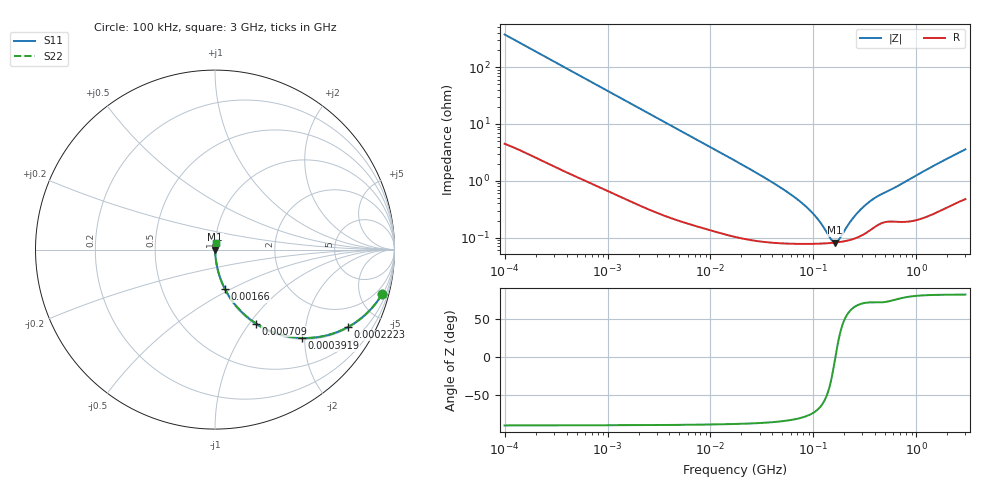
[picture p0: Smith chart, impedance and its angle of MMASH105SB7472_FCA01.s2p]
! MMASH105SB7472_FCA01  S-PARAMETER MODEL  ( Standard Model )
! Model Generated by TAIYO YUDEN Corporation (http://www.ty-top.com)
! Version 1.0
! TAIYO YUDEN Control No. 220601
! Copyright(c) 2019 TAIYO YUDEN CO.,LTD. All Rights Reserved.
! Product Description (link to TY-COMPAS)
! https://ds.yuden.co.jp/TYCOMPAS/or/detail?pn=MMASH105SB7472KFCA01&u=M
! Products Name : Multilayer Ceramic Capacitors
! Characteristics :
!  Capacitance : 4700 [pF] , Rated Voltage : 100 [V] , TCC : X7R
!  Case Size : 1.0 x 0.5 / 0.039 x 0.02 [mm/inch] , Thickness : 0.5 / 0.02 [mm/inch]
!  (Conditions: Temperature = 25 [degC] , DC Bias Voltage = 0 [V])
! External Node Assignments :
!  1  o---| |---o  2
! GND o---------o GND
! Frequency Range : 100kHz  -  3GHz  [ 401 STEP ]
# MHZ S RI R 50
! Freq[MHz].  S11 Real  S11 Imag  S21 Real  S21 Imag  S12 Real  S12 Imag  S22 Real  S22 Imag
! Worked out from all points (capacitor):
!   401 points, 100 kHz to 3 GHz, reference 50 ohm
!   read as one part in series: C = 4.23 nF near 105.3 kHz
!   lowest |Z| = 81.9 mohm at 163.1 MHz (marker M1)
!   series resonance near 163.6 MHz, so ESL is about 220 pH
!   S11 on the Smith chart (normalised r, x): 100 kHz: 1.09, -7.50; 222.3 kHz: 1.05, -3.40; 391.9 kHz: 1.03, -1.94; 709 kHz: 1.02, -1.08; 1.66 MHz: 1.01, -0.46; 3 GHz: 1.01, +0.07
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0.1  0.9311 -0.2474  0.0689 0.2474  0.0689 0.2474  0.9311 -0.2474
0.151038  0.8582 -0.3424  0.1418 0.3424  0.1418 0.3424  0.8582 -0.3424
0.222319  0.74 -0.4319  0.26 0.4319  0.26 0.4319  0.74 -0.4319
0.391939  0.4844 -0.4924  0.5156 0.4924  0.5156 0.4924  0.4844 -0.4924
0.562235  0.3173 -0.4577  0.6827 0.4577  0.6827 0.4577  0.3173 -0.4577
0.709011  0.2285 -0.4118  0.7715 0.4118  0.7715 0.4118  0.2285 -0.4118
1.043626  0.1232 -0.32  0.8768 0.32  0.8768 0.32  0.1232 -0.32
1.659646  0.0548 -0.2184  0.9452 0.2184  0.9452 0.2184  0.0548 -0.2184
3.161081  0.0173 -0.1202  0.9827 0.1202  0.9827 0.1202  0.0173 -0.1202
17.7727  0.0015 -0.0219  0.9985 0.0219  0.9985 0.0219  0.0015 -0.0219
53.83243  0.00083 -0.00658  0.9992 0.00658  0.9992 0.00658  0.00083 -0.00658
75.25761  0.000793 -0.00417  0.9992 0.00417  0.9992 0.00417  0.000793 -0.00417
97.38194  0.000784 -0.00264  0.9992 0.00264  0.9992 0.00264  0.000784 -0.00264
116.6348  0.000787 -0.00168  0.9992 0.00168  0.9992 0.00168  0.000787 -0.00168
147.0833  0.000804 -0.000521  0.9992 0.000521  0.9992 0.000521  0.000804 -0.000521
163.0551  0.000818 -1.6e-05  0.9992 1.6e-05  0.9992 1.6e-05  0.000818 -1.6e-05
176.1623  0.000832 0.000363  0.9992 -0.000363  0.9992 -0.000363  0.000832 0.000363
233.9019  0.000927 0.0018  0.9991 -0.0018  0.9991 -0.0018  0.000927 0.0018
302.6647  0.00113 0.00321  0.9989 -0.00321  0.9989 -0.00321  0.00113 0.00321
391.6425  0.00154 0.00469  0.9985 -0.00469  0.9985 -0.00469  0.00154 0.00469
547.5153  0.00196 0.0065  0.998 -0.0065  0.998 -0.0065  0.00196 0.0065
3000  0.00597 0.035  0.994 -0.035  0.994 -0.035  0.00597 0.035
